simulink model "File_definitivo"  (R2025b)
settings: Solver=FixedStepAuto  StartTime=0.0  StopTime=25  FixedStep=0.0002  RelTol=1e-3  EnableMultiTasking=on
InitFcn:
  | np=8;
  | ke=0.0404;
  | wn=5600/60*2*pi;
  | Tn=0.134; %Nm
  | B=Tn*0.1/wn;
  | inertia=19.01e-6; %kgm2
  | kfan=(Tn*0.9)/wn/wn;
  | prescalertim5=1;
  | 
  | offset1=2125;
  | offset2=2128;
  | offset3=2119;
  | 
  | gain1=0.015;
  | gain2=gain1;
  | gain3=gain1;
  | 
  | kp_i = 0.1505*4;
  | ki_i = 286.5*4;
  | 
  | V_dc = 20;
  | cpt=2048;
undefined symbols (not defined in the file): Based, DiscIntNeverNeededParam, STM32H5xx
libraries: stm32f4xxblockslib x5, mcbeeMathTransformLib x4, slpidlib x3, stm32h5xxblockslib x3, stm32blockslib x2, simulink x2

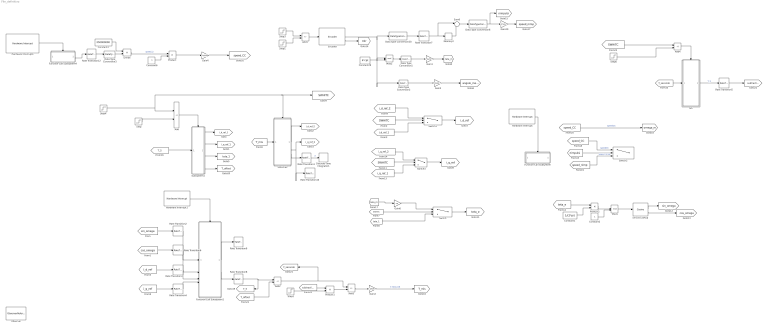
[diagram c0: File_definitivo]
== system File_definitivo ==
  Add : Sum  Inputs=-+
  Add1 : Sum  Inputs=-+
  Add2 : Sum  Inputs=+-
  Add3 : Sum  Inputs=+-
  Add4 : Sum  Inputs=+-
  Constant1 : Constant  Value=1/(2*pi)
  Constant2 : Constant
  Constant29 : Constant  Value=4*cpt  OutDataTypeStr=uint32
  Constant3 : Constant  Commented=on  Value=250000000  OutDataTypeStr=double  SampleTime=-1
  Constant6 : Constant  Commented=on  OutDataTypeStr=double  SampleTime=0.001
  Data Type Conversion1 : DataTypeConversion  OutDataTypeStr=double
  Data Type Conversion2 : DataTypeConversion  OutDataTypeStr=int32
  Data Type Conversion20 : DataTypeConversion  OutDataTypeStr=int32
  Data Type Conversion3 : DataTypeConversion  Commented=on  OutDataTypeStr=double
  Data Type Conversion6 : DataTypeConversion  OutDataTypeStr=double
  Discrete-Time Integrator1 : DiscreteIntegrator  SampleTime=-1  ICPrevOutput=DiscIntNeverNeededParam  ICPrevScaledInput=DiscIntNeverNeededParam
  Divide : Product  Commented=on  Inputs=*/
  Encoder : stm32blockslib/Encoder  TimerModule=TIM2  EnableResetInput=on  OutputDirection=on  SampleTime=-1
  Function-Call Subsystem : Subsystem  TreatAsAtomicUnit=on
  Function-Call Subsystem1 : Subsystem  TreatAsAtomicUnit=on
  Function-Call Subsystem4 : Subsystem  Commented=on  TreatAsAtomicUnit=on
  Gain1 : Gain  Gain=2*pi/(4*cpt)
  Gain2 : Gain  Gain=3.3/4096/101.7*(22.695/(2.0042*3.3/1000))
  Gain20 : Gain  Gain=(2*pi/(4*cpt))/0.001
  Gain3 : Gain  Gain=2*pi/(4*cpt)/156
  Gain4 : Gain  Commented=on  Gain=2*pi/cpt
  Gain6 : Gain  Gain=np
  Hardware Interrupt : stm32h5xxblockslib/Hardware Interrupt  ISRGroup=Timer (TIM)  ISRName=TIM8_UP_IRQHandler  ISRNumber=81  EventsList={ 'on', 'TIM8 Update', '1'; 'off', 'Custom event', '2' }  SelectedEvents={'TIM8 Update'}  TaskPriority=30  DisablePreemption=off  ClearInterruptFlagsAtEndOfEvent=off  InterruptDefinitionFile=$(TARGET_ROOT)/registry/interrupts/STM32U5xxBased_interrupts.xml  HardwareBoard=STM32H5xx Based  EnableSimPort=off
  Hardware Interrupt1 : stm32h5xxblockslib/Hardware Interrupt  ISRGroup=Analog to digital converter (ADC)  ISRName=ADC1_IRQHandler  ISRNumber=52  EventsList={ 'off', 'ADC1 OVR', '1'; 'off', 'ADC1 Reg EoCS', '2'; 'on', 'ADC1 Inj EoCS', '3'; 'off', 'ADC1 Inj JQOVF', '4'; 'off', 'ADC1 Watchdog1', '5'; 'off', 'ADC1 Watchdog2', '6'; 'off', 'ADC1 Watchdog3', '7'; 'off', 'Custom event', '8' }  SelectedEvents={'ADC1 Inj EoCS'}  TaskPriority=30  DisablePreemption=off  ClearInterruptFlagsAtEndOfEvent=off  InterruptDefinitionFile=$(TARGET_ROOT)/registry/interrupts/STM32U5xxBased_interrupts.xml  HardwareBoard=STM32H5xx Based  EnableSimPort=off
  Hardware Interrupt4 : stm32h5xxblockslib/Hardware Interrupt  Commented=on  ISRGroup=Timer (TIM)  ISRName=TIM5_IRQHandler  ISRNumber=63  EventsList={ 'off', 'TIM5 Update', '1'; 'on', 'TIM5 CC1', '2'; 'off', 'TIM5 CC2', '3'; 'off', 'TIM5 CC3', '4'; 'off', 'TIM5 CC4', '5'; 'off', 'TIM5 Trigger', '6'; 'off', 'TIM5 DIR', '7'; 'off', 'TIM5 IDX', '8'; 'off', 'TIM5 IERR', '9'; 'off', 'TIM5 TERR', '10'; 'off', 'Custom event', '11' }  SelectedEvents={'TIM5 CC1'}  TaskPriority=29  DisablePreemption=off  ClearInterruptFlagsAtEndOfEvent=off  InterruptDefinitionFile=$(TARGET_ROOT)/registry/interrupts/STM32U5xxBased_interrupts.xml  HardwareBoard=STM32H5xx Based  EnableSimPort=off
  Memory2 : Memory  InheritSampleTime=on
  Mod1 : Math  Operator=mod
  Mod2 : Math  Operator=mod  OutputSignalType=real
  Observer : ObserverReference  ObserverModelName=Maxon_0902_forzometro_Observer1
  Product : Product  Commented=on
  Product1 : Product
  Product2 : Product
  Rate Transition1 : RateTransition  Deterministic=off  OutPortSampleTime=0.001
  Rate Transition10 : RateTransition  Deterministic=off  OutPortSampleTime=0.001
  Rate Transition12 : RateTransition  Commented=on  Integrity=off  OutPortSampleTime=0.001
  Rate Transition{2..6,8} (6 alike) : RateTransition  Deterministic=off
  Rate Transition7 : RateTransition  OutPortSampleTime=0.001
  Rate Transition9 : RateTransition  Deterministic=off  OutPortSampleTime=0.001
  SiS : Subsystem
  SinCos Lookup : simulink/Lookup Tables/Cosine  Formula=sin(2*pi*u) and cos(2*pi*u)  NumDataPoints=(2^5)+1  OutputWordLength=16  InternalRulePriority=Speed
  Sistema2 : Subsystem
  Step : Step  Time=5  SampleTime=0
  Step1 : Step  Time=7  SampleTime=0
  Step2 : Step  Time=21
  Step3 : Step  Time=7.01  SampleTime=0
  Step4 : Step  Time=10  SampleTime=0
  Step6 : Step  Time=11  SampleTime=0
  Subsystem1 : Subsystem
  Sum6 : Sum  Inputs=|+-
  Switch : Switch  Threshold=0.5
  Switch1 : Switch  Threshold=0.5
  Switch2 : Switch  Commented=on  Threshold=55
  Switch3 : Switch  Threshold=0.5
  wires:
  Switch2/1 -> ?
  Data Type Conversion3/1 -> Divide/2
  Encoder/2 -> [Dir]
  Constant1/1 -> Product2/2
  [T_5] -> Subsystem1/1(In1)
  Hardware Interrupt4/1 -> Function-Call Subsystem4/Trigger
  Product1/1 -> Add3/2
  Step6/1 -> Add4/2
  [i_q_ref_1] -> Switch3/3
  Constant2/1 -> Mod1/2
  Constant3/1 -> Divide/1
  [SWHITC] -> Switch/2
  Gain3/1 -> [angolo_mecc]
  Step2/1 -> Product1/2
  Add3/1 -> Gain2/1
  Divide/1 -> Product/1  "speed_2"
  SinCos Lookup/1 -> [sin_omega]
  Memory2/1 -> Sum6/2
  Subsystem1/3(Out3) -> [teta_1]
  Rate Transition12/1 -> Data Type Conversion3/1
  Subsystem1/1(Out1) -> [i_d_ref_1]
  Switch3/1 -> [i_q_ref]
  Gain2/1 -> [T_mis]  "T_filtro_IIR"
  Data Type Conversion6/1 -> Gain20/1, [nimpulsi]
  [teta_m] -> Gain6/1
  [speed_nimp] -> Switch2/3  "speed_nimp"
  [speed_CC] -> Switch2/1  "speedCC"
  [teta_e] -> Product2/1
  Constant6/1 -> Product/2
  Add1/1 -> Encoder/1
  Subsystem1/4(Out5) -> [T_offset]
  Rate Transition5/1 -> [subtraction]
  [subtraction] -> Product1/1
  [SWHITC] -> Switch1/2
  Step4/1 -> [SWHITC], Sistema2/Enable, Add/1
  Product2/1 -> Mod1/1
  [SWHITC] -> Switch3/2
  [SWHITC] -> Add4/1
  Rate Transition3/1 -> Function-Call Subsystem1/3(In8)
  Rate Transition2/1 -> Function-Call Subsystem1/1(In1)
  Gain1/1 -> [teta_m]
  Encoder/1 -> Data Type Conversion2/1, Mod2/1, Data Type Conversion20/1
  [teta_1] -> Switch/3
  Mod1/1 -> SinCos Lookup/1
  Gain6/1 -> Switch/1
  Add2/1 -> Add3/1, [T_secondo]
  [speed_CC] -> [omega_m]  "speedCC"
  Hardware Interrupt/1 -> Function-Call Subsystem/Trigger
  Data Type Conversion1/1 -> Gain1/1
  [T_secondo] -> SiS/1(In2)
  Switch/1 -> [teta_e]
  Switch1/1 -> [i_d_ref]
  [T_offset] -> Add2/2
  [i_d_ref_2] -> Switch1/1
  [i_q_ref] -> Rate Transition4/1
  [nimpulsi] -> Switch2/2
  SinCos Lookup/2 -> [cos_omega]
  Function-Call Subsystem4/2(Out3) -> Rate Transition12/1
  Gain20/1 -> [speed_nimp]
  Hardware Interrupt1/1 -> Function-Call Subsystem1/Trigger
  Data Type Conversion2/1 -> Gain3/1
  SiS/1(Out4) -> Rate Transition5/1  "T_2"
  Data Type Conversion20/1 -> Rate Transition7/1
  Rate Transition4/1 -> Function-Call Subsystem1/4(In9)
  Constant29/1 -> Mod2/2
  Step1/1 -> Add1/2
  Rate Transition1/1 -> Discrete-Time Integrator1/1  "e"
  Subsystem1/2(Out2) -> [i_q_ref_1]
  Product/1 -> Gain4/1
  [cos_omega] -> Rate Transition6/1
  [sin_omega] -> Rate Transition2/1
  Rate Transition6/1 -> Function-Call Subsystem1/2(In2)
  Sum6/1 -> Data Type Conversion6/1
  Gain4/1 -> [speed_CC]
  [T_mis] -> Sistema2/1(In1)
  Function-Call Subsystem1/2(Out3) -> Rate Transition8/1
  Sistema2/1(Out1) -> [i_d_ref_2]
  Function-Call Subsystem1/1(Out1) -> Rate Transition9/1
  Rate Transition8/1 -> [T_5], Add2/1
  Mod2/1 -> Data Type Conversion1/1
  [i_q_ref_2] -> Switch3/1
  Rate Transition7/1 -> Memory2/1, Sum6/1
  Sistema2/2(Out2) -> Rate Transition10/1, [i_q_ref_2]
  Add4/1 -> SiS/Enable
  Add/1 -> Subsystem1/Enable
  [i_d_ref_1] -> Switch1/3
  Step/1 -> Add/2
  Step3/1 -> Add1/1
  [i_d_ref] -> Rate Transition3/1
  Sistema2/3(Out3) -> Rate Transition1/1

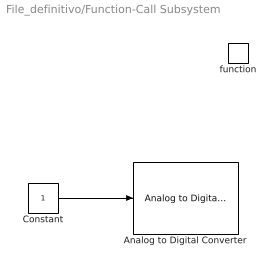
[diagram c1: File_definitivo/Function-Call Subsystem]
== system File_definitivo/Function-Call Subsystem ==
  function : TriggerPort  TriggerType=function-call  VariantControl=(inherit)
  Analog to Digital Converter : stm32f4xxblockslib/Analog to Digital Converter  ADCModule=ADC1  ConversionGroup=Injected  TriggerMode=Trigger only  NumberOfConversions=1  EnableBufferConv=off  BufferLength=1  OutputStatus=off  SampleTime=-1  EnableSimPort=off  hoistedMaskSrc=ECSoC/ECSimCodegen/Analog to Digital Converter
  Constant : Constant  OutDataTypeStr=boolean
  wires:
  Constant/1 -> Analog to Digital Converter/1

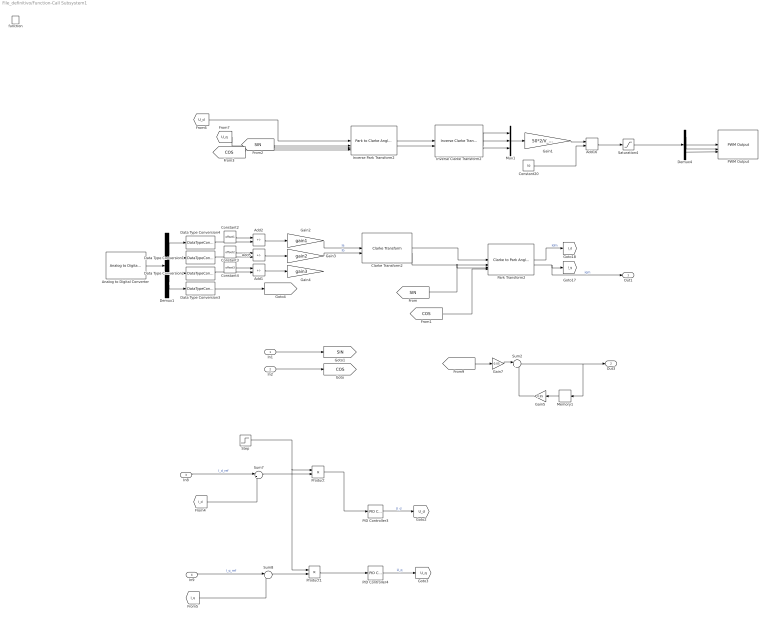
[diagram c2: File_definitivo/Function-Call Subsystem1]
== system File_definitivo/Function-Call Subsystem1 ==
  In1 : Inport
  In2 : Inport  Port=2
  In8 : Inport  Port=3
  In9 : Inport  Port=4
  function : TriggerPort  TriggerType=function-call  VariantControl=(inherit)
  Add1 : Sum  Inputs=-+
  Add16 : Sum
  Add2 : Sum  Inputs=-+
  Add5 : Sum  Inputs=-+
  Analog to Digital Converter : stm32f4xxblockslib/Analog to Digital Converter  ADCModule=ADC1  ConversionGroup=Injected  TriggerMode=Read results only  NumberOfConversions=4  EnableBufferConv=off  BufferLength=1  OutputStatus=off  SampleTime=-1  EnableSimPort=off  hoistedMaskSrc=ECSoC/ECSimCodegen/Analog to Digital Converter
  Clarke Transform2 : mcbeeMathTransformLib/Clarke Transform  VariantControl=Variant2  PowerInvariant=on  UseWithEmbedded=on  PhaseInput=Two inputs
  Constant2 : Constant  Value=offset1
  Constant20 : Constant  Value=50
  Constant3 : Constant  Value=offset2
  Constant4 : Constant  Value=offset3
  Data Type Conversion{1..4} (4 alike) : DataTypeConversion  OutDataTypeStr=double
  Demux1 : Demux
  Demux4 : Demux  Outputs=3
  Gain1 : Gain  Gain=50*2/V_dc
  Gain2 : Gain  Gain=gain1
  Gain3 : Gain  Gain=gain2
  Gain4 : Gain  Gain=gain3
  Gain5 : Gain  Gain=0.95
  Gain7 : Gain  Gain=0.05
  Inverse Clarke Transform2 : mcbeeMathTransformLib/Inverse Clarke Transform  PowerInvariant=on  UseWithEmbedded=on  PhaseInput=Two inputs
  Inverse Park Transform2 : mcbeeMathTransformLib/Park to Clarke Angle Transform  AxisAlignment=D-axis  UseWithEmbedded=on  PhaseInput=Two inputs  ThetaInput=Sine and Cosine electrical position  AngleInput=Per-unit  N_points=1024
  Memory1 : Memory  InheritSampleTime=on
  Mux1 : Mux  Inputs=3
  PID Controller3 : slpidlib/PID Controller  Controller=PI  Form=Parallel  TimeDomain=Discrete-time  UseExternalTs=off  SampleTime=-1  IntegratorMethod=Forward Euler  FilterMethod=Forward Euler  ControllerParametersSource=internal  P=kp_i  I=ki_i  UseKiTs=off  D=0  UseExternalDerivativeSource=off  N=100  UseFilter=on  TunerSelectOption=Transfer Function Based (PID Tuner App)  InitialConditionSource=internal  InitialConditionForIntegrator=0  InitialConditionForFilter=0  DifferentiatorICPrevScaledInput=0  ExternalReset=none  TrackingMode=off  Kt=1  LimitOutput=on  SatLimitsSource=internal  UpperSaturationLimit=V_dc/sqrt(2)  LowerSaturationLimit=-V_dc/sqrt(2)  LinearizeAsGain=on  AntiWindupMode=clamping  Kb=1  LimitIntegrator=off  UpperIntegratorSaturationLimit=inf  LowerIntegratorSaturationLimit=-inf  POutMin=[]  POutMax=[]  IOutMin=[]  IOutMax=[]  DOutMin=[]  DOutMax=[]  NOutMin=[]  NOutMax=[]  SumOutMin=[]  SumOutMax=[]  SaturationOutMin=[]  SaturationOutMax=[]  PParamMin=[]  PParamMax=[]  IParamMin=[]  IParamMax=[]  DParamMin=[]  DParamMax=[]  NParamMin=[]  NParamMax=[]  KbParamMin=[]  KbParamMax=[]  KtParamMin=[]  KtParamMax=[]  KbOutMin=[]  KbOutMax=[]  KtOutMin=[]  KtOutMax=[]  IntegratorOutMin=[]  IntegratorOutMax=[]  FilterOutMin=[]  FilterOutMax=[]  SumI1OutMin=[]  SumI1OutMax=[]  SumI2OutMin=[]  SumI2OutMax=[]  SumI3OutMin=[]  SumI3OutMax=[]  SumI4OutMin=[]  SumI4OutMax=[]  SumDOutMin=[]  SumDOutMax=[]  DifferentiatorOutMin=[]  DifferentiatorOutMax=[]  FilterDiffOutCoefMin=[]  FilterDiffOutCoefMax=[]  ReciprocalOutMin=[]  ReciprocalOutMax=[]  SumDenOutMin=[]  SumDenOutMax=[]  SumNumOutMin=[]  SumNumOutMax=[]  DivideOutMin=[]  DivideOutMax=[]  UdiffTsProdOutMin=[]  UdiffTsProdOutMax=[]  NTsProdOutMin=[]  NTsProdOutMax=[]  UintegralTsProdOutMin=[]  UintegralTsProdOutMax=[]  UngainTsProdOutMin=[]  UngainTsProdOutMax=[]  ClampingZeroOutDataTypeStr=Inherit: Inherit via back propagation  ClampingZeroOutMin=[]  ClampingZeroOutMax=[]  FilterDenConstantOutDataTypeStr=Inherit: Inherit via back propagation  FilterDenConstantOutMin=[]  FilterDenConstantOutMax=[]  PCopyOutDataTypeStr=Inherit: Inherit via back propagation  PCopyOutMin=[]  PCopyOutMax=[]  NCopyOutDataTypeStr=Inherit: Inherit via back propagation  NCopyOutMin=[]  NCopyOutMax=[]  IntegratorContinuousStateAttributes=''  IntegratorStateMustResolveToSignalObject=off  IntegratorRTWStateStorageClass=Auto  FilterContinuousStateAttributes=''  FilterStateMustResolveToSignalObject=off  FilterRTWStateStorageClass=Auto  ParallelPVariant=InternalParameters  IdealPVariant=Disabled  IVariant=InternalParameters  DVariant=Disabled  IntegratorVariant=Discrete  SatVariant=Enabled  AWVariant=DiscClampingParallel  PCopyVariant=Disabled  TRVariant=Disabled  FdbkBlocksVariant=Forward  IdealPFdbkVariant=Disabled  SatFdbkVariant=Disabled  DerivativeFilterVariant=Disabled  NVariant=Disabled  NCopyVariant=Disabled_SignalSpec  FilterICVariant=Disabled  IntegratorICVariant=InternalICs  ExternalResetVariant=Disabled  TRSumVariant=Passthrough  SumFdbkVariant=Disabled  SumVariant=Sum_PI  TsampFilterVariant=InternalTs  TsampNgainVariant=Passthrough  TsampIntegralVariant=Disabled_SignalSpec  ExternalSaturationOutDataTypeStr=Inherit: Same as second input  DerivativeSourceVariant=Disabled  PreIntVariant=InternalPreInt
  PID Controller4 : slpidlib/PID Controller  Controller=PI  Form=Parallel  TimeDomain=Discrete-time  UseExternalTs=off  SampleTime=-1  IntegratorMethod=Forward Euler  FilterMethod=Forward Euler  ControllerParametersSource=internal  P=kp_i  I=ki_i  UseKiTs=off  D=0  UseExternalDerivativeSource=off  N=100  UseFilter=on  TunerSelectOption=Transfer Function Based (PID Tuner App)  InitialConditionSource=internal  InitialConditionForIntegrator=0  InitialConditionForFilter=0  DifferentiatorICPrevScaledInput=0  ExternalReset=none  TrackingMode=off  Kt=1  LimitOutput=on  SatLimitsSource=internal  UpperSaturationLimit=V_dc/sqrt(2)  LowerSaturationLimit=-V_dc/sqrt(2)  LinearizeAsGain=on  AntiWindupMode=clamping  Kb=1  LimitIntegrator=off  UpperIntegratorSaturationLimit=inf  LowerIntegratorSaturationLimit=-inf  POutMin=[]  POutMax=[]  IOutMin=[]  IOutMax=[]  DOutMin=[]  DOutMax=[]  NOutMin=[]  NOutMax=[]  SumOutMin=[]  SumOutMax=[]  SaturationOutMin=[]  SaturationOutMax=[]  PParamMin=[]  PParamMax=[]  IParamMin=[]  IParamMax=[]  DParamMin=[]  DParamMax=[]  NParamMin=[]  NParamMax=[]  KbParamMin=[]  KbParamMax=[]  KtParamMin=[]  KtParamMax=[]  KbOutMin=[]  KbOutMax=[]  KtOutMin=[]  KtOutMax=[]  IntegratorOutMin=[]  IntegratorOutMax=[]  FilterOutMin=[]  FilterOutMax=[]  SumI1OutMin=[]  SumI1OutMax=[]  SumI2OutMin=[]  SumI2OutMax=[]  SumI3OutMin=[]  SumI3OutMax=[]  SumI4OutMin=[]  SumI4OutMax=[]  SumDOutMin=[]  SumDOutMax=[]  DifferentiatorOutMin=[]  DifferentiatorOutMax=[]  FilterDiffOutCoefMin=[]  FilterDiffOutCoefMax=[]  ReciprocalOutMin=[]  ReciprocalOutMax=[]  SumDenOutMin=[]  SumDenOutMax=[]  SumNumOutMin=[]  SumNumOutMax=[]  DivideOutMin=[]  DivideOutMax=[]  UdiffTsProdOutMin=[]  UdiffTsProdOutMax=[]  NTsProdOutMin=[]  NTsProdOutMax=[]  UintegralTsProdOutMin=[]  UintegralTsProdOutMax=[]  UngainTsProdOutMin=[]  UngainTsProdOutMax=[]  ClampingZeroOutDataTypeStr=Inherit: Inherit via back propagation  ClampingZeroOutMin=[]  ClampingZeroOutMax=[]  FilterDenConstantOutDataTypeStr=Inherit: Inherit via back propagation  FilterDenConstantOutMin=[]  FilterDenConstantOutMax=[]  PCopyOutDataTypeStr=Inherit: Inherit via back propagation  PCopyOutMin=[]  PCopyOutMax=[]  NCopyOutDataTypeStr=Inherit: Inherit via back propagation  NCopyOutMin=[]  NCopyOutMax=[]  IntegratorContinuousStateAttributes=''  IntegratorStateMustResolveToSignalObject=off  IntegratorRTWStateStorageClass=Auto  FilterContinuousStateAttributes=''  FilterStateMustResolveToSignalObject=off  FilterRTWStateStorageClass=Auto  ParallelPVariant=InternalParameters  IdealPVariant=Disabled  IVariant=InternalParameters  DVariant=Disabled  IntegratorVariant=Discrete  SatVariant=Enabled  AWVariant=DiscClampingParallel  PCopyVariant=Disabled  TRVariant=Disabled  FdbkBlocksVariant=Forward  IdealPFdbkVariant=Disabled  SatFdbkVariant=Disabled  DerivativeFilterVariant=Disabled  NVariant=Disabled  NCopyVariant=Disabled_SignalSpec  FilterICVariant=Disabled  IntegratorICVariant=InternalICs  ExternalResetVariant=Disabled  TRSumVariant=Passthrough  SumFdbkVariant=Disabled  SumVariant=Sum_PI  TsampFilterVariant=InternalTs  TsampNgainVariant=Passthrough  TsampIntegralVariant=Disabled_SignalSpec  ExternalSaturationOutDataTypeStr=Inherit: Same as second input  DerivativeSourceVariant=Disabled  PreIntVariant=InternalPreInt
  PWM Output : stm32f4xxblockslib/PWM Output  ProcessorFamily=STM32G4  TimerModule=TIM8  DutycycleUnits=Percentage  EnableChannel1=on  EnableCaptureCompare1Input=off  EnableCaptureCompare1ComplementaryInput=off  EnableOutputCompare1ModeInput=off  EnableChannel2=on  EnableCaptureCompare2Input=off  EnableCaptureCompare2ComplementaryInput=off  EnableOutputCompare2ModeInput=off  EnableChannel3=on  EnableCaptureCompare3Input=off  EnableCaptureCompare3ComplementaryInput=off  EnableOutputCompare3ModeInput=off  EnableChannel4=off  EnableCaptureCompare4Input=off  EnableCaptureCompare4ComplementaryInput=off  EnableOutputCompare4ModeInput=off  EnableChannel5=off  EnableCaptureCompare5Input=off  EnableOutputCompare5ModeInput=off  EnableChannel6=off  EnableCaptureCompare6Input=off  EnableOutputCompare6ModeInput=off  EnableCounterInput=off  EnableMainOutputInput=off  EnableFrequencyInput=off  SetRCAfterCE=off  OutputDirection=off  OutputMainOutputEnableStatus=off  SampleTime=0.1  EnableSimPort=off  EnableUpdateEvent=off  EnableCaptureCompare1Event=off  EnableCaptureCompare2Event=off  EnableCaptureCompare3Event=off  EnableCaptureCompare4Event=off  EnableTriggerEvent=off  EnableBreakEvent=off  EnableBreakEvent2=off  hoistedMaskSrc=ECSoC/ECSimCodegen/PWM Output
  Park Transform2 : mcbeeMathTransformLib/Clarke to Park Angle Transform  AxisAlignment=D-axis  UseWithEmbedded=on  PhaseInput=Two inputs  ThetaInput=Sine and Cosine electrical position  AngleInput=Per-unit  N_points=1024
  Product : Product
  Product1 : Product
  Saturation4 : Saturate  UpperLimit=99  LowerLimit=1
  Step : Step  Time=5
  Sum2 : Sum  Inputs=|++
  Sum7 : Sum  Inputs=|+-
  Sum8 : Sum  Inputs=|+-
  Out1 : Outport
  Out3 : Outport  Port=2
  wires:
  Constant2/1 -> Add2/1
  Saturation4/1 -> Demux4/1
  Demux4/3 -> PWM Output/3
  Gain1/1 -> Add16/1
  Inverse Park Transform2/1 -> Inverse Clarke Transform2/1
  Demux1/4 -> Data Type Conversion3/1
  Gain2/1 -> Clarke Transform2/1  "Ia"
  [SIN] -> Inverse Park Transform2/3
  Add1/1 -> Gain4/1
  Clarke Transform2/1 -> Park Transform2/1
  Analog to Digital Converter/1 -> Demux1/1
  Add2/1 -> Gain2/1
  Clarke Transform2/2 -> Park Transform2/2
  Demux4/2 -> PWM Output/2
  Demux4/1 -> PWM Output/1
  Inverse Clarke Transform2/2 -> Mux1/2
  [COS] -> Inverse Park Transform2/4
  Mux1/1 -> Gain1/1
  Data Type Conversion1/1 -> Add5/2
  Demux1/3 -> Data Type Conversion2/1
  Data Type Conversion2/1 -> Add1/2
  Constant4/1 -> Add1/1
  Constant20/1 -> Add16/2
  Demux1/1 -> Data Type Conversion4/1
  Add5/1 -> Gain3/1
  Inverse Clarke Transform2/1 -> Mux1/1
  Inverse Park Transform2/2 -> Inverse Clarke Transform2/2
  Constant3/1 -> Add5/1
  Gain3/1 -> Clarke Transform2/2  "Ib"
  Demux1/2 -> Data Type Conversion1/1
  Inverse Clarke Transform2/3 -> Mux1/3
  Data Type Conversion4/1 -> Add2/2
  In2/1 -> [COS]
  In1/1 -> [SIN]
  [SIN] -> Park Transform2/3
  [COS] -> Park Transform2/4
  Sum7/1 -> Product/2
  In8/1 -> Sum7/1  "I_d_ref"
  In9/1 -> Sum8/1  "I_q_ref"
  Product1/1 -> PID Controller4/1
  Sum8/1 -> Product1/2
  Product/1 -> PID Controller3/1
  Step/1 -> Product1/1, Product/1
  Park Transform2/1 -> [I_d]  "Idm"
  Park Transform2/2 -> Out1/1, [I_q]  "iqm"
  [I_d] -> Sum7/2
  [I_q] -> Sum8/2
  PID Controller3/1 -> [U_d]  "U_d"
  PID Controller4/1 -> [U_q]  "U_q"
  [U_d] -> Inverse Park Transform2/1
  [U_q] -> Inverse Park Transform2/2
  Add16/1 -> Saturation4/1
  Data Type Conversion3/1 -> [T]
  Sum2/1 -> Out3/1, Memory1/1
  [T] -> Gain7/1
  Memory1/1 -> Gain5/1
  Gain5/1 -> Sum2/2
  Gain7/1 -> Sum2/1

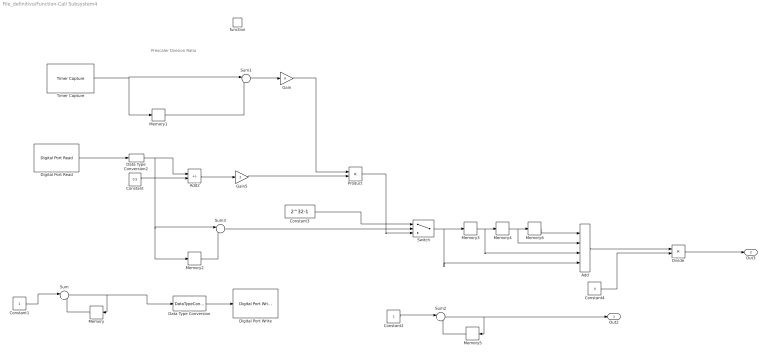
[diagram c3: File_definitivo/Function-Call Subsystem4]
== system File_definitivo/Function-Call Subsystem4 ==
  note: Prescaler Division Ratio
  function : TriggerPort  TriggerType=function-call  VariantControl=(inherit)
  Add : Sum  Inputs=++++
  Add2 : Sum  Inputs=+-
  Constant : Constant  Value=0.5
  Constant1 : Constant  Commented=on  OutDataTypeStr=uint8  SampleTime=-1
  Constant2 : Constant  OutDataTypeStr=uint8  SampleTime=-1
  Constant3 : Constant  Value=2^32-1
  Constant4 : Constant  Value=4
  Data Type Conversion : DataTypeConversion  Commented=on  OutDataTypeStr=boolean
  Data Type Conversion2 : DataTypeConversion  OutDataTypeStr=double
  Digital Port Read : stm32f4xxblockslib/Digital Port Read  PortName=GPIOB  PinNumber=[3]  ReadOperation=on  IOAsArray=on  SampleTime=-1  EnableSimPort=off  hoistedMaskSrc=ECSoC/ECSimCodegen/Digital Port Read
  Digital Port Write : stm32f4xxblockslib/Digital Port Write  Commented=on  PortName=GPIOA  PinNumber=[6]  ReadOperation=off  IOAsArray=on  EnableSimPort=off  hoistedMaskSrc=ECSoC/ECSimCodegen/Digital Port Write
  Divide : Product  Inputs=*/
  Gain : Gain
  Gain5 : Gain  Gain=2
  Memory : Memory  Commented=on  InheritSampleTime=on
  Memory{1..6} (6 alike) : Memory  InheritSampleTime=on
  Product : Product
  Sum : Sum  Commented=on  Inputs=|+-
  Sum1 : Sum  Inputs=|+-
  Sum2 : Sum  Inputs=|+-
  Sum3 : Sum  Inputs=|+-
  Switch : Switch  Criteria=u2 ~= 0
  Timer Capture : stm32blockslib/Timer Capture  TimerModule=TIM5  SelectedChannel=CH1  CaptureLength=1  OutputDataLength=off  OutputOverrunStatus=off  OutputDirection=off  SampleTime=-1
  Out2 : Outport
  Out3 : Outport  Port=2
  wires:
  Memory/1 -> Sum/2
  Constant1/1 -> Sum/1
  Data Type Conversion/1 -> Digital Port Write/1
  Sum/1 -> Memory/1, Data Type Conversion/1
  Timer Capture/1 -> Memory1/1, Sum1/1
  Sum1/1 -> Gain/1
  Sum2/1 -> Out2/1, Memory5/1
  Constant2/1 -> Sum2/1
  Memory5/1 -> Sum2/2
  Data Type Conversion2/1 -> Sum3/1, Memory2/1, Add2/1
  Constant/1 -> Add2/2
  Gain5/1 -> Product/2
  Add2/1 -> Gain5/1
  Gain/1 -> Product/1
  Digital Port Read/1 -> Data Type Conversion2/1
  Memory1/1 -> Sum1/2
  Product/1 -> Switch/3
  Memory2/1 -> Sum3/2
  Sum3/1 -> Switch/2
  Constant3/1 -> Switch/1
  Switch/1 -> Add/4, Memory3/1
  Memory3/1 -> Add/3, Memory4/1
  Memory4/1 -> Add/2, Memory6/1
  Memory6/1 -> Add/1
  Add/1 -> Divide/1
  Divide/1 -> Out3/1
  Constant4/1 -> Divide/2

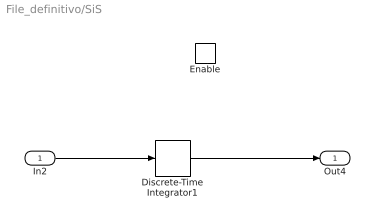
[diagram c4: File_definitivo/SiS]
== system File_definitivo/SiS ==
  In2 : Inport
  Enable : EnablePort
  Discrete-Time Integrator1 : DiscreteIntegrator  SampleTime=-1  ICPrevOutput=DiscIntNeverNeededParam  ICPrevScaledInput=DiscIntNeverNeededParam
  Out4 : Outport
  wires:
  In2/1 -> Discrete-Time Integrator1/1
  Discrete-Time Integrator1/1 -> Out4/1

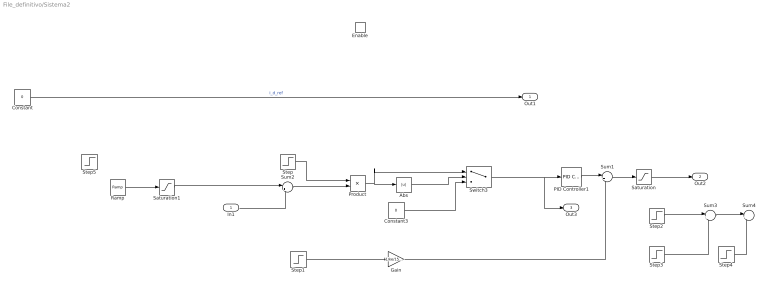
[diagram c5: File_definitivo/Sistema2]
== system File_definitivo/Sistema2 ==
  In1 : Inport
  Enable : EnablePort
  Abs : Abs
  Constant : Constant  Value=0
  Constant3 : Constant  Value=0
  Gain : Gain  Gain=1/ke/156*1*2
  PID Controller1 : slpidlib/PID Controller  Controller=PID  Form=Parallel  TimeDomain=Discrete-time  UseExternalTs=off  SampleTime=-1  IntegratorMethod=Forward Euler  FilterMethod=Forward Euler  ControllerParametersSource=internal  P=1.5  I=14  UseKiTs=off  D=1/100*1.5  UseExternalDerivativeSource=off  N=100  UseFilter=off  TunerSelectOption=Transfer Function Based (PID Tuner App)  InitialConditionSource=internal  InitialConditionForIntegrator=0  InitialConditionForFilter=0  DifferentiatorICPrevScaledInput=0  ExternalReset=none  TrackingMode=off  Kt=1  LimitOutput=on  SatLimitsSource=internal  UpperSaturationLimit=3.3  LowerSaturationLimit=-3.3  LinearizeAsGain=on  AntiWindupMode=clamping  Kb=1  LimitIntegrator=off  UpperIntegratorSaturationLimit=inf  LowerIntegratorSaturationLimit=-inf  POutMin=[]  POutMax=[]  IOutMin=[]  IOutMax=[]  DOutMin=[]  DOutMax=[]  NOutMin=[]  NOutMax=[]  SumOutMin=[]  SumOutMax=[]  SaturationOutMin=[]  SaturationOutMax=[]  PParamMin=[]  PParamMax=[]  IParamMin=[]  IParamMax=[]  DParamMin=[]  DParamMax=[]  NParamMin=[]  NParamMax=[]  KbParamMin=[]  KbParamMax=[]  KtParamMin=[]  KtParamMax=[]  KbOutMin=[]  KbOutMax=[]  KtOutMin=[]  KtOutMax=[]  IntegratorOutMin=[]  IntegratorOutMax=[]  FilterOutMin=[]  FilterOutMax=[]  SumI1OutMin=[]  SumI1OutMax=[]  SumI2OutMin=[]  SumI2OutMax=[]  SumI3OutMin=[]  SumI3OutMax=[]  SumI4OutMin=[]  SumI4OutMax=[]  SumDOutMin=[]  SumDOutMax=[]  DifferentiatorOutMin=[]  DifferentiatorOutMax=[]  FilterDiffOutCoefMin=[]  FilterDiffOutCoefMax=[]  ReciprocalOutMin=[]  ReciprocalOutMax=[]  SumDenOutMin=[]  SumDenOutMax=[]  SumNumOutMin=[]  SumNumOutMax=[]  DivideOutMin=[]  DivideOutMax=[]  UdiffTsProdOutMin=[]  UdiffTsProdOutMax=[]  NTsProdOutMin=[]  NTsProdOutMax=[]  UintegralTsProdOutMin=[]  UintegralTsProdOutMax=[]  UngainTsProdOutMin=[]  UngainTsProdOutMax=[]  ClampingZeroOutDataTypeStr=Inherit: Inherit via back propagation  ClampingZeroOutMin=[]  ClampingZeroOutMax=[]  FilterDenConstantOutDataTypeStr=Inherit: Inherit via back propagation  FilterDenConstantOutMin=[]  FilterDenConstantOutMax=[]  PCopyOutDataTypeStr=Inherit: Inherit via back propagation  PCopyOutMin=[]  PCopyOutMax=[]  NCopyOutDataTypeStr=Inherit: Inherit via back propagation  NCopyOutMin=[]  NCopyOutMax=[]  IntegratorContinuousStateAttributes=''  IntegratorStateMustResolveToSignalObject=off  IntegratorRTWStateStorageClass=Auto  FilterContinuousStateAttributes=''  FilterStateMustResolveToSignalObject=off  FilterRTWStateStorageClass=Auto  ParallelPVariant=InternalParameters  IdealPVariant=Disabled  IVariant=InternalParameters  DVariant=InternalParameters  IntegratorVariant=Discrete  SatVariant=Enabled  AWVariant=DiscClampingParallel  PCopyVariant=Disabled  TRVariant=Disabled  FdbkBlocksVariant=Forward  IdealPFdbkVariant=Disabled  SatFdbkVariant=Disabled  DerivativeFilterVariant=Differentiator  NVariant=Passthrough  NCopyVariant=Disabled_SignalSpec  FilterICVariant=InternalICsDifferentiator  IntegratorICVariant=InternalICs  ExternalResetVariant=Disabled  TRSumVariant=Passthrough  SumFdbkVariant=Disabled  SumVariant=Sum_PID  TsampFilterVariant=InternalTs  TsampNgainVariant=Passthrough  TsampIntegralVariant=Disabled_SignalSpec  ExternalSaturationOutDataTypeStr=Inherit: Same as second input  DerivativeSourceVariant=ErrorSignal  PreIntVariant=InternalPreInt
  Product : Product
  Ramp : simulink/Sources/Ramp  slope=100  start=23  InitialOutput=0
  Saturation : Saturate  UpperLimit=3.3  LowerLimit=-3.3
  Saturation1 : Saturate  UpperLimit=1  LowerLimit=0
  Step : Step  Time=23  SampleTime=0
  Step1 : Step  Time=23  SampleTime=0
  Step2 : Step  Time=22  SampleTime=0
  Step3 : Step  Time=23  After=0.9  SampleTime=0
  Step4 : Step  Time=25  SampleTime=0
  Step5 : Step  Time=23  SampleTime=0
  Sum1 : Sum  Inputs=|++
  Sum2 : Sum  Inputs=|+-
  Sum3 : Sum  Inputs=|+-
  Sum4 : Sum  Inputs=|++
  Switch3 : Switch  Threshold=0.07
  Out1 : Outport
  Out2 : Outport  Port=2
  Out3 : Outport  Port=3
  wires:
  Constant/1 -> Out1/1  "i_d_ref"
  Ramp/1 -> Saturation1/1
  PID Controller1/1 -> Sum1/1
  Sum2/1 -> Product/2
  Step/1 -> Product/1
  In1/1 -> Sum2/2
  Product/1 -> Switch3/1, Abs/1
  Switch3/1 -> PID Controller1/1, Out3/1
  Constant3/1 -> Switch3/3
  Abs/1 -> Switch3/2
  Sum1/1 -> Saturation/1
  Step2/1 -> Sum3/1
  Sum3/1 -> Sum4/1
  Step3/1 -> Sum3/2
  Sum4/1 -> ?
  Step4/1 -> Sum4/2
  Saturation/1 -> Out2/1
  Step1/1 -> Gain/1
  Saturation1/1 -> Sum2/1
  Gain/1 -> Sum1/2

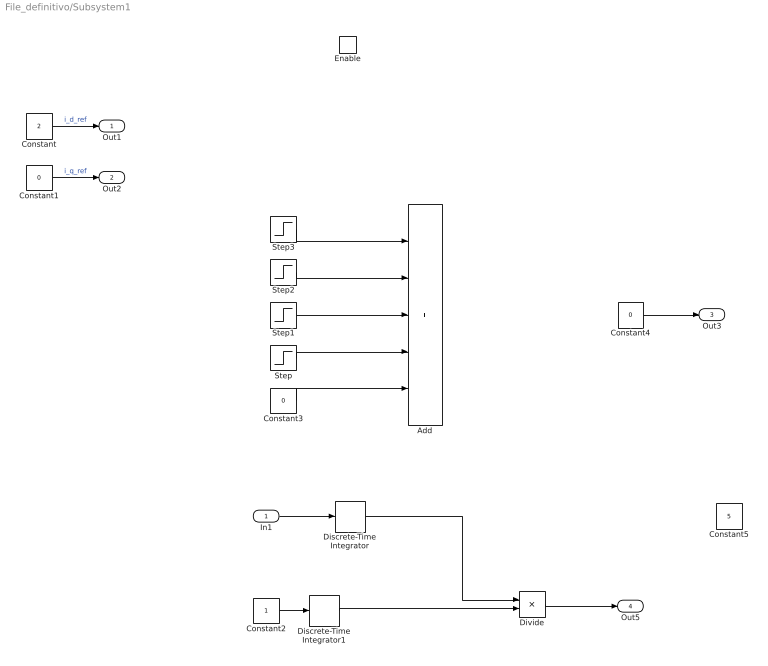
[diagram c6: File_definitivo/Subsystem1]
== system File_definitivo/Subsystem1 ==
  In1 : Inport
  Enable : EnablePort
  Add : Sum  Commented=on  Inputs=+++++
  Constant : Constant  Value=2
  Constant1 : Constant  Value=0
  Constant2 : Constant
  Constant3 : Constant  Commented=on  Value=0
  Constant4 : Constant  Value=0
  Constant5 : Constant  Value=5
  Discrete-Time Integrator : DiscreteIntegrator  SampleTime=-1  ICPrevOutput=DiscIntNeverNeededParam  ICPrevScaledInput=DiscIntNeverNeededParam
  Discrete-Time Integrator1 : DiscreteIntegrator  SampleTime=-1  ICPrevOutput=DiscIntNeverNeededParam  ICPrevScaledInput=DiscIntNeverNeededParam
  Divide : Product  Inputs=*/
  Step : Step  Commented=on  Time=10  After=pi/2  SampleTime=0
  Step1 : Step  Commented=on  Time=11  After=pi/2  SampleTime=0
  Step2 : Step  Commented=on  Time=12  After=pi/2  SampleTime=0
  Step3 : Step  Commented=on  Time=13  After=pi/2  SampleTime=0
  Out1 : Outport
  Out2 : Outport  Port=2
  Out3 : Outport  Port=3
  Out5 : Outport  Port=4
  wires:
  Constant/1 -> Out1/1  "i_d_ref"
  Constant1/1 -> Out2/1  "i_q_ref"
  Step2/1 -> Add/2
  Step/1 -> Add/4
  Step1/1 -> Add/3
  Constant3/1 -> Add/5
  Step3/1 -> Add/1
  Add/1 -> ?  "Teta"
  Constant4/1 -> Out3/1
  In1/1 -> Discrete-Time Integrator/1
  Discrete-Time Integrator/1 -> Divide/1
  Discrete-Time Integrator1/1 -> Divide/2
  Divide/1 -> Out5/1
  Constant2/1 -> Discrete-Time Integrator1/1
